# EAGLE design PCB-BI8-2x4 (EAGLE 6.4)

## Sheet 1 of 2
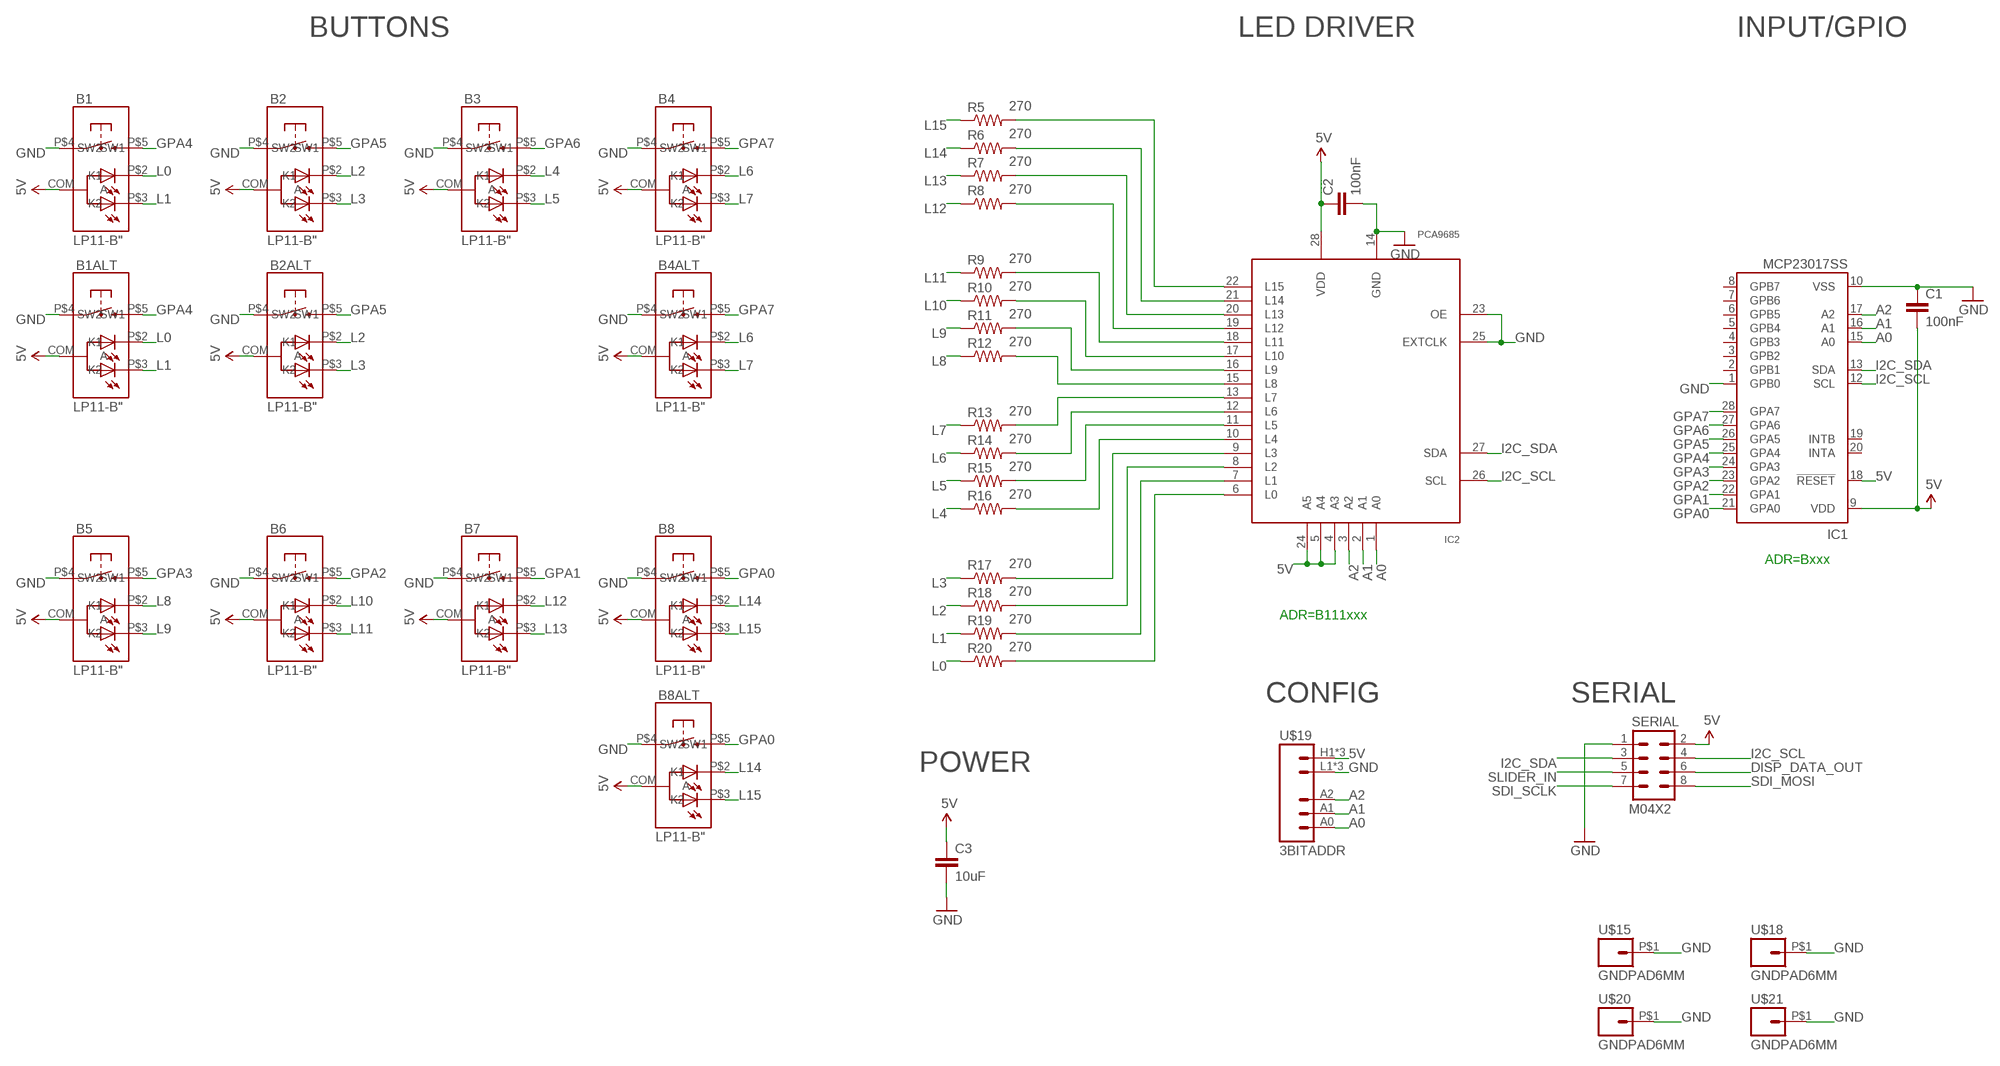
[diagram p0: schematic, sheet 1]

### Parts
B1  LP11-B"  [LP11]
B1ALT  LP11-B"  [LP11]
B2  LP11-B"  [LP11]
B2ALT  LP11-B"  [LP11]
B3  LP11-B"  [LP11]
B4  LP11-B"  [LP11]
B4ALT  LP11-B"  [LP11]
B5  LP11-B"  [LP11]
B6  LP11-B"  [LP11]
B7  LP11-B"  [LP11]
B8  LP11-B"  [LP11]
B8ALT  LP11-B"  [LP11]
C1  100nF  CAP0603-CAP  [0603-CAP]
C2  100nF  CAP0603-CAP  [0603-CAP]
C3  10uF  CAP0805  [0805]
IC1  MCP23017SS  [SSOP28]
IC2  PCA9685  [TSSOP28]
R5  270  RESISTOR0603-RES  [0603-RES]
R6  270  RESISTOR0603-RES  [0603-RES]
R7  270  RESISTOR0603-RES  [0603-RES]
R8  270  RESISTOR0603-RES  [0603-RES]
R9  270  RESISTOR0603-RES  [0603-RES]
R10  270  RESISTOR0603-RES  [0603-RES]
R11  270  RESISTOR0603-RES  [0603-RES]
R12  270  RESISTOR0603-RES  [0603-RES]
R13  270  RESISTOR0603-RES  [0603-RES]
R14  270  RESISTOR0603-RES  [0603-RES]
R15  270  RESISTOR0603-RES  [0603-RES]
R16  270  RESISTOR0603-RES  [0603-RES]
R17  270  RESISTOR0603-RES  [0603-RES]
R18  270  RESISTOR0603-RES  [0603-RES]
R19  270  RESISTOR0603-RES  [0603-RES]
R20  270  RESISTOR0603-RES  [0603-RES]
SERIAL  M04X2  [2X4]
U$15  GNDPAD6MM  [3.2MMPAD6MM]
U$18  GNDPAD6MM  [3.2MMPAD6MM]
U$19  3BITADDR  [3BITADDR]
U$20  GNDPAD6MM  [3.2MMPAD6MM]
U$21  GNDPAD6MM  [3.2MMPAD6MM]

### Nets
5V [Power]: B1.COM(A) B1ALT.COM(A) B2.COM(A) B2ALT.COM(A) B3.COM(A) B4.COM(A) B4ALT.COM(A) B5.COM(A) B6.COM(A) B7.COM(A) B8.COM(A) B8ALT.COM(A) C1.2 C2.1 C3.1 IC1.9(VDD) IC1.18(!RESET) IC2.4(A3) IC2.5(A4) IC2.24(A5) IC2.28(VDD) SERIAL.2 U$19.H1(VCC) U$19.H2(VCC) U$19.H3(VCC)
A0: IC1.15(A0) IC2.1(A0) U$19.A0
A1: IC1.16(A1) IC2.2(A1) U$19.A1
A2: IC1.17(A2) IC2.3(A2) U$19.A2
DISP_DATA_OUT: SERIAL.6
GND [Power]: B1.P$4(SW1) B1ALT.P$4(SW1) B2.P$4(SW1) B2ALT.P$4(SW1) B3.P$4(SW1) B4.P$4(SW1) B4ALT.P$4(SW1) B5.P$4(SW1) B6.P$4(SW1) B7.P$4(SW1) B8.P$4(SW1) B8ALT.P$4(SW1) C1.1 C2.2 C3.2 IC1.1(GPB0) IC1.10(VSS) IC2.14(GND) IC2.23(OE) IC2.25(EXTCLK) SERIAL.1 U$15.P$1 U$18.P$1 U$19.L1(GND) U$19.L2(GND) U$19.L3(GND) U$20.P$1 U$21.P$1
GPA0: B8.P$5(SW2) B8ALT.P$5(SW2) IC1.21(GPA0)
GPA1: B7.P$5(SW2) IC1.22(GPA1)
GPA2: B6.P$5(SW2) IC1.23(GPA2)
GPA3: B5.P$5(SW2) IC1.24(GPA3)
GPA4: B1.P$5(SW2) B1ALT.P$5(SW2) IC1.25(GPA4)
GPA5: B2.P$5(SW2) B2ALT.P$5(SW2) IC1.26(GPA5)
GPA6: B3.P$5(SW2) IC1.27(GPA6)
GPA7: B4.P$5(SW2) B4ALT.P$5(SW2) IC1.28(GPA7)
I2C_SCL: IC1.12(SCL) IC2.26(SCL) SERIAL.4
I2C_SDA: IC1.13(SDA) IC2.27(SDA) SERIAL.3
L0: B1.P$2(K1) B1ALT.P$2(K1) R20.1
L1: B1.P$3(K2) B1ALT.P$3(K2) R19.1
L2: B2.P$2(K1) B2ALT.P$2(K1) R18.1
L3: B2.P$3(K2) B2ALT.P$3(K2) R17.1
L4: B3.P$2(K1) R16.1
L5: B3.P$3(K2) R15.1
L6: B4.P$2(K1) B4ALT.P$2(K1) R14.1
L7: B4.P$3(K2) B4ALT.P$3(K2) R13.1
L8: B5.P$2(K1) R12.1
L9: B5.P$3(K2) R11.1
L10: B6.P$2(K1) R10.1
L11: B6.P$3(K2) R9.1
L12: B7.P$2(K1) R8.1
L13: B7.P$3(K2) R7.1
L14: B8.P$2(K1) B8ALT.P$2(K1) R6.1
L15: B8.P$3(K2) B8ALT.P$3(K2) R5.1
N$4: IC2.13(L7) R13.2
N$5: IC2.12(L6) R14.2
N$7: IC2.11(L5) R15.2
N$9: IC2.10(L4) R16.2
N$10: IC2.9(L3) R17.2
N$11: IC2.8(L2) R18.2
N$12: IC2.7(L1) R19.2
N$19: IC2.6(L0) R20.2
N$20: IC2.15(L8) R12.2
N$21: IC2.16(L9) R11.2
N$22: IC2.17(L10) R10.2
N$23: IC2.18(L11) R9.2
N$24: IC2.19(L12) R8.2
N$25: IC2.20(L13) R7.2
N$26: IC2.21(L14) R6.2
N$27: IC2.22(L15) R5.2
SDI_MOSI: SERIAL.8
SDI_SCLK: SERIAL.7
SLIDER_IN: SERIAL.5
Unconnected: IC1.2(GPB1) IC1.3(GPB2) IC1.4(GPB3) IC1.5(GPB4) IC1.6(GPB5) IC1.7(GPB6) IC1.8(GPB7) IC1.19(INTB) IC1.20(INTA)

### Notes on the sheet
- BUTTONS | LED DRIVER | INPUT/GPIO
- ADR=Bxxx
- ADR=B111xxx
- CONFIG | SERIAL
- POWER

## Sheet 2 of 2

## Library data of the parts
B1 B1ALT B2 B2ALT B3 B4 B4ALT B5-B8 B8ALT = SKAARHOJ:LP11-B
C1-C3 = SparkFun:CAP: Capacitor
IC1 = microchip:MCP23017: http://ww1.microchip.com/downloads/en/DeviceDoc/21952a.pdf Source: http://ww1.microchip.com/downloads/en/DeviceDoc/21952a.pdf; MF: MICROCHIP; MPN: MCP23017-E/SS; OC_FARNELL: 1467674; OC_NEWARK: 31K2960
IC2 = wsmith:PCA9685
R5-R20 = SparkFun:RESISTOR: Resistor
SERIAL = SparkFun:M04X2
U$15 U$18 U$20 U$21 = SKAARHOJ:GNDPAD
U$19 = SKAARHOJ:3BITADDR

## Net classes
0 default: width 0.203 mm, drill 0.406 mm, clearance 0.203 mm
1 Power: width 0.406 mm, drill 0.61 mm, clearance 0.203 mm

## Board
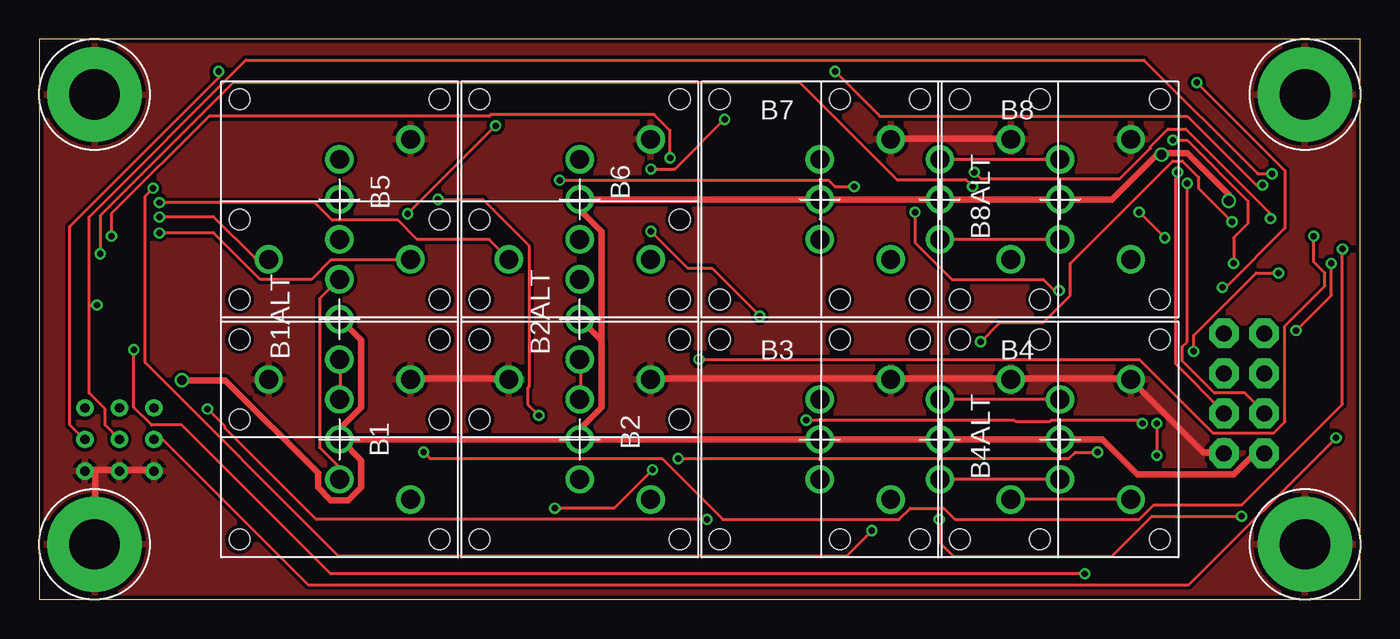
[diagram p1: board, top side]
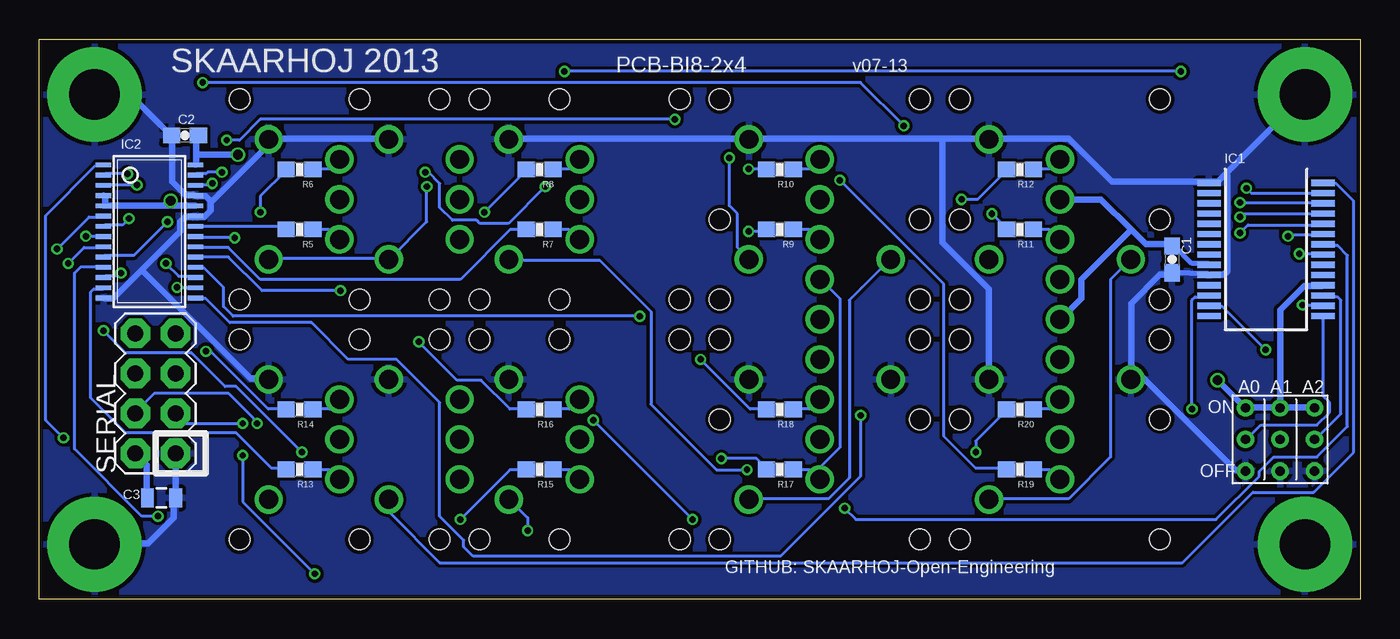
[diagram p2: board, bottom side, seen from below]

Size 83.82 x 35.56 mm. Coordinates in mm from the lower left corner, seen from the top.
Outline: 0,0 83.82,0 83.82,35.56 0,35.56 0,0
Copper layers (1*16): Top 0.035mm / dielectric 1.5mm / Bottom 0.035mm
Design rules "Fusion_eagle_rule_v1.1": minimum track width 6mil, minimum drill 12mil, track to track 6mil, track to pad 6mil, pad to pad 6mil, via to via 6mil, smd to smd 0mil, copper to edge 10mil, drill to drill 10mil, minimum pad ring 10mil, minimum via ring 6mil, stop-mask expansion 2mil, vias tented up to drill 100mil, thermal gap 10mil

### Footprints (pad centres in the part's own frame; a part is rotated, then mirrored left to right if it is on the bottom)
LP11 = drill 1.2: COM 0,0; P$2 0,2.54; P$3 0,-2.54; P$4 4.5,3.81; P$5 4.5,-3.81 | hole 1.3: -6.35,6.35; 6.35,6.35; 6.35,-6.35; -6.35,-6.35
0603-CAP = smd 1.1 x 1: 1 -0.85,0; 2 0.85,0
0805 = smd 0.8 x 1.2: 1 -0.9,0; 2 0.9,0
SSOP28 = smd 0.4 x 1.5: 1 -4.225,-3.625; 2 -3.575,-3.625; 3 -2.925,-3.625; 4 -2.275,-3.625; 5 -1.625,-3.625; 6 -0.975,-3.625; 7 -0.325,-3.625; 8 0.325,-3.625; 9 0.975,-3.625; 10 1.625,-3.625; 11 2.275,-3.625; 12 2.925,-3.625; 13 3.575,-3.625; 14 4.225,-3.625; 15 4.225,3.625; 16 3.575,3.625; 17 2.925,3.625; 18 2.275,3.625; 19 1.625,3.625; 20 0.975,3.625; 21 0.325,3.625; 22 -0.325,3.625; 23 -0.975,3.625; 24 -1.625,3.625; 25 -2.275,3.625; 26 -2.925,3.625; 27 -3.575,3.625; 28 -4.225,3.625
TSSOP28 = smd 0.305 x 0.991: 1 -4.225,-2.918; 2 -3.575,-2.918; 3 -2.925,-2.918; 4 -2.275,-2.918; 5 -1.625,-2.918; 6 -0.975,-2.918; 7 -0.325,-2.918; 8 0.325,-2.918; 9 0.975,-2.918; 10 1.625,-2.918; 11 2.275,-2.918; 12 2.925,-2.918; 13 3.575,-2.918; 14 4.225,-2.918; 15 4.225,2.918; 16 3.575,2.918; 17 2.925,2.918; 18 2.275,2.918; 19 1.625,2.918; 20 0.975,2.918; 21 0.325,2.918; 22 -0.325,2.918; 23 -0.975,2.918; 24 -1.625,2.918; 25 -2.275,2.918; 26 -2.925,2.918; 27 -3.575,2.918; 28 -4.225,2.918
0603-RES = smd 1.1 x 1: 1 -0.85,0; 2 0.85,0
2X4 = drill 1.016 pad 1.88 octagon: 1 -3.81,-1.27; 2 -3.81,1.27; 3 -1.27,-1.27; 4 -1.27,1.27; 5 1.27,-1.27; 6 1.27,1.27; 7 3.81,-1.27; 8 3.81,1.27
3.2MMPAD6MM = drill 3.2 pad 6: P$1 0,0
3BITADDR = drill 0.6: A0 -2.2,0; A1 0,0; A2 2.2,0; H1 -2.2,2; H2 0,2; H3 2.2,2; L1 -2.2,-2; L2 0,-2; L3 2.2,-2

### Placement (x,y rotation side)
B1  19.05,10.16 0 top
B1ALT  19.05,17.78 180 top
B2  34.29,10.16 0 top
B2ALT  34.29,17.78 180 top
B3  49.53,10.16 0 top
B4  64.77,10.16 0 top
B4ALT  57.15,10.16 0 top
B5  19.05,25.4 0 top
B6  34.29,25.4 0 top
B7  49.53,25.4 0 top
B8  64.77,25.4 0 top
B8ALT  57.15,25.4 0 top
C1  11.94,21.59 90 bottom
C2  74.57,29.46 180 bottom
C3  76.07,6.45 0 bottom
IC1  5.97,22.23 270 bottom
IC2  76.83,23.37 270 bottom
R5  67.31,23.5 180 bottom
R6  67.31,27.3 180 bottom
R7  52.07,23.5 180 bottom
R8  52.07,27.3 180 bottom
R9  36.83,23.5 180 bottom
R10  36.83,27.3 180 bottom
R11  21.59,23.5 180 bottom
R12  21.59,27.3 180 bottom
R13  67.31,8.26 180 bottom
R14  67.31,12.06 180 bottom
R15  52.07,8.26 180 bottom
R16  52.07,12.06 180 bottom
R17  36.83,8.26 180 bottom
R18  36.83,12.06 180 bottom
R19  21.59,8.26 180 bottom
R20  21.59,12.06 180 bottom
SERIAL  76.45,13.08 90 bottom
U$15  3.5,3.5 0 top
U$18  80.32,3.5 0 top
U$19  5.08,10.16 0 bottom
U$20  3.5,32.06 0 top
U$21  80.32,32.06 0 top

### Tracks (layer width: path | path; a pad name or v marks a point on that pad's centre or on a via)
5V  (via drill 0.61)
  Top 0.406: v75.49,25.3 75.49,25.7 72.85,28.35 71.32,28.35 v71.22,28.25 70.92,28.25 68.07,25.4 B8.COM B8ALT.COM B7.COM B6.COM 34.34,25.4 34.34,24.69 35.66,23.37 35.66,16.66 35.56,16.56 | SERIAL.2 77.72,9.25 77.11,9.25 75.79,7.92 69.7,7.92 67.46,10.16 B4.COM B4ALT.COM B3.COM B2.COM | 35.56,16.56 34.34,17.78 B2ALT.COM | 35.56,16.56 35.66,16.46 35.66,12.19 34.34,10.87 34.34,10.16 B2.COM | B1.COM 19.1,10.16 19.1,10.87 20.42,12.19 20.42,16.46 19.1,17.78 B1ALT.COM | v9.04,13.92 11.79,13.92 17.68,8.03 17.68,7.11 18.49,6.3 19.61,6.3 20.42,7.11 20.42,8.84 19.2,10.06 B1.COM | B1.COM B2.COM
  Bottom 0.305: IC1.9 9.68,21.34 10.67,21.34 11.77,22.44 C1.2
  Bottom 0.406: 79.65,24.99 75.49,24.99 | 75.49,24.99 73.97,24.99 IC2.24 | 79.65,24.99 IC2.5 | 79.65,24.99 79.65,25.6 IC2.4 | 73.86,28.25 73.86,29.36 73.76,29.46 C2.1 | 73.86,28.25 73.86,27.64 IC2.28 | v71.22,28.25 73.86,28.25 | v75.49,25.3 75.49,24.99 | C3.1 77.01,6.5 77.01,8.53 77.72,9.25 SERIAL.2 | U$19.H2 5.08,18.39 3.56,19.91 2.44,19.91 IC1.18 | U$19.H3 2.95,12.19 4.98,12.19 U$19.H2 | U$19.H2 5.28,12.19 7.21,12.19 U$19.H1 7.42,12.29 v9.04,13.92 | 14.53,23.47 16.46,25.4 B5.COM | 14.53,23.47 13.61,22.55 11.99,22.55 C1.2 | 14.53,23.47 17.68,20.32 17.68,19.1 19,17.78 B1ALT.COM
A0  (via drill 0.41)
  Top 0.203: v82.3,10.26 72.95,0.91 17.07,0.91 7.82,10.16 U$19.A0
  Bottom 0.203: v82.3,10.26 83.41,11.38 83.41,24.38 80.26,27.53 79.76,27.53 IC2.1 | IC1.15 2.34,17.98 2.34,12.9 1.93,12.5 1.93,11.89 2.74,11.07 6.3,11.07 7.21,10.16 U$19.A0
A1  (via drill 0.41)
  Top 0.203: v78.23,27.03 77.32,27.03 70.1,34.24 13.11,34.24 3.15,24.28 3.15,18.69 | 3.15,18.69 3.15,13.11 4.17,12.09 4.17,11.07 U$19.A1 | 3.15,18.69 v3.66,18.69
  Bottom 0.203: v78.23,27.03 79.65,27.03 IC2.2 | v3.66,18.69 2.44,18.69 IC1.16
A2  (via drill 0.41)
  Top 0.203: v77.62,26.31 77.22,26.31 72.85,30.68 53.34,30.68 v50.49,33.53 | v11.38,33.53 11.38,33.12 1.93,23.67 1.93,11.07 2.85,10.16 U$19.A2
  Bottom 0.203: v77.62,26.31 79.65,26.31 IC2.3 | v11.38,33.53 v50.49,33.53 | IC1.17 2.34,19.2 1.42,19.2 1.22,19 1.22,11.79 2.85,10.16 U$19.A2
GND
  Top 0.406: B2.P$4 38.81,14.02 53.95,14.02 B3.P$4 54.15,14.02 61.57,14.02 B4ALT.P$4 61.77,14.02 69.19,14.02 B4.P$4 69.39,13.82 73.86,9.35 75.18,9.35 SERIAL.1 | 3.56,8.23 5.08,8.23 U$19.L2 5.18,8.23 7.21,8.23 U$19.L1 | 3.56,8.23 2.95,8.23 U$19.L3 | 3.56,8.23 3.56,3.56 U$15.P$1 | B1.P$4 23.57,14.02 29.77,14.02 B2ALT.P$4 | B7.P$4 54.05,29.26 61.57,29.26 B8ALT.P$4
  Bottom 0.305: IC1.10 9.7,20.7 10.79,20.7 10.83,20.74 C1.1
  Bottom 0.406: SERIAL.1 75.18,6.5 C3.2 75.29,6.3 75.29,5.18 76.91,3.56 80.26,3.56 U$18.P$1 | U$20.P$1 8.53,27.03 | 8.53,27.03 9.04,26.52 9.55,26.52 IC1.1 9.75,26.52 15.75,26.52 18.49,29.26 23.37,29.26 B5.P$4 23.57,29.26 26.52,29.26 | IC1.10 9.45,20.62 8.64,20.62 8.43,20.83 8.43,26.92 8.53,27.03 | C1.1 11.99,20.62 12.7,20.62 14.53,18.8 14.53,14.02 B1ALT.P$4 14.43,14.73 7.92,8.23 7.32,8.23 U$19.L1 | 26.52,29.26 38.71,29.26 B6.P$4 38.91,29.26 53.95,29.26 B7.P$4 | 26.52,29.26 26.52,22.66 23.57,19.71 23.57,14.02 B1.P$4 | 72.95,25.3 72.95,24.69 73.36,24.28 73.86,24.28 IC2.23 74.07,24.28 74.57,24.28 74.88,23.98 74.88,23.37 77.32,20.93 | 72.95,25.3 73.25,25.6 73.86,25.6 IC2.25 74.07,25.7 74.57,25.7 75.39,26.52 75.39,29.46 C2.2 75.59,29.57 78.03,32 80.26,32 U$21.P$1 | 77.32,20.93 79.15,19.1 79.65,19.1 IC2.14 | 72.95,25.3 72.85,25.3 69.29,28.85 69.29,29.16 B8.P$4 69.09,29.26 61.67,29.26 B8ALT.P$4 | 77.32,20.93 70.41,14.02 69.29,14.02 B4.P$4
  pour Top: 0,0 83.82,0 83.82,35.56 0,35.56
  pour Bottom: 0,0 83.82,0 83.82,35.56 0,35.56
GPA0  (via drill 0.41)
  Top 0.203: v3.86,21.95 3.86,24.38 12.29,32.82 48.26,32.82 54.46,26.62 58.83,26.62 v59.23,26.21
  Bottom 0.203: v3.86,21.95 2.44,21.95 IC1.21 | v59.23,26.21 59.23,23.98 61.57,21.64 B8ALT.P$5 61.67,21.64 69.19,21.64 B8.P$5
GPA1  (via drill 0.41)
  Top 0.203: v32.72,5.79 36.47,5.79 v38.91,8.23
  Bottom 0.203: v32.72,5.79 32,5.08 9.14,5.08 6.4,7.82 6.4,8.13 5.49,9.04 2.74,9.04 0.81,10.97 0.81,21.84 1.42,22.45 2.34,22.45 IC1.22 | v38.91,8.23 40.84,8.23 45.01,12.39 45.01,18.29 48.26,21.54 53.95,21.54 B7.P$5
GPA2  (via drill 0.41)
  Top 0.203: v4.57,23.06 4.57,24.49 10.77,30.68 28.55,30.68 28.65,30.79 39.01,30.79 40.03,29.77 v40.03,28.04
  Bottom 0.203: v4.57,23.06 4.47,23.16 2.44,23.16 IC1.23 | v40.03,28.04 40.03,24.99 39.52,24.49 39.52,22.35 38.81,21.64 B6.P$5
GPA3  (via drill 0.41)
  Top 0.203: v7.62,23.27 11.07,23.27 14.02,20.32 17.27,20.32 18.49,21.54 23.47,21.54 B5.P$5
  Bottom 0.203: v7.62,23.27 7.11,23.77 2.44,23.77 IC1.24
GPA4  (via drill 0.41)
  Top 0.203: v7.62,24.28 11.07,24.28 13.72,21.64 14.53,21.64 B1ALT.P$5
  Bottom 0.203: v7.62,24.28 7.42,24.49 2.44,24.49 IC1.25 | B1.P$5 23.47,6.4 18.49,6.4 15.85,9.04 15.85,20.32 14.63,21.54 B1ALT.P$5
GPA5  (via drill 0.41)
  Top 0.203: v7.62,25.2 17.48,25.2 18.59,24.08 22.76,24.08 23.98,22.86 28.55,22.86 29.77,21.64 B2ALT.P$5
  Bottom 0.203: v7.62,25.2 2.44,25.2 IC1.26 | B2.P$5 38.71,6.4 33.73,6.4 32.41,7.72 32.41,19 29.87,21.54 B2ALT.P$5
GPA6  (via drill 0.41)
  Top 0.203: v7.21,26.11 6.71,25.6 6.71,15.04 19,2.74 51.21,2.74 v52.83,4.37
  Bottom 0.203: v7.21,26.11 6.91,25.81 2.44,25.81 IC1.27 | v52.83,4.37 52.83,5.18 53.95,6.3 B3.P$5
GPA7
  Top 0.203: B4.P$5 69.19,6.4 61.67,6.4 B4ALT.P$5
  Bottom 0.203: IC1.28 2.34,26.42 1.52,26.42 0.41,25.3 0.41,9.35 2.95,6.81 6.81,6.81 11.28,2.34 58.42,2.34 61.57,5.49 61.57,6.3 B4ALT.P$5
I2C_SCL  (via drill 0.41)
  Top 0.203: v72.85,26.42 72.85,16.36 72.54,16.05 72.54,15.14 74.57,13.11 76.5,13.11 77.72,11.89 SERIAL.4 | v10.67,12.09 11.79,10.97 11.79,10.87 17.58,5.08 v42.37,5.08 | v48.67,11.38 61.87,11.38 61.98,11.28 64.11,11.28 64.21,11.38 69.8,11.38 v70,11.18
  Bottom 0.203: v72.85,26.42 72.95,26.31 73.86,26.31 IC2.26 | v10.67,12.09 10.67,19 10.46,19.2 9.65,19.2 IC1.12 | v48.67,11.38 v42.37,5.08 | v70,11.18 70.21,11.38 70.21,11.48 71.83,13.11 76.5,13.11 77.72,11.89 SERIAL.4
I2C_SDA  (via drill 0.41)
  Top 0.203: v72.24,27.13 72.24,26.82 72.14,26.72 72.14,14.94 75.18,11.89 SERIAL.3 | v5.99,15.85 5.99,12.19 7.11,11.07 9.04,11.07 18.49,1.63 v66.34,1.63 | v70.92,11.18 v70.92,9.14
  Bottom 0.203: v72.24,27.13 73.15,27.13 73.25,27.03 73.86,27.03 IC2.27 | v5.99,15.85 8.74,18.59 9.55,18.59 IC1.13 | v66.34,1.63 70.92,6.2 v70.92,9.14 | v70.92,11.18 74.57,11.18 75.18,11.79 SERIAL.3
L0
  Top 0.203: B1.P$2 19.1,12.7 19.1,15.24 B1ALT.P$2
  Bottom 0.203: R20.1 20.73,12.09 19.71,12.09 19.1,12.7 B1.P$2
L1
  Top 0.203: B1.P$3 19,7.62 19,8.43 17.78,9.65 17.78,19.1 19,20.32 B1ALT.P$3
  Bottom 0.203: R19.1 20.73,8.23 19.71,8.23 19.1,7.62 B1.P$3
L2
  Top 0.203: B2.P$2 34.34,12.7 34.34,15.24 B2ALT.P$2
  Bottom 0.203: R18.1 35.97,12.09 34.95,12.09 34.34,12.7 B2.P$2
L3
  Bottom 0.203: R17.1 35.97,8.23 34.95,8.23 34.34,7.62 B2.P$3 34.65,8.03 33.02,9.65 33.02,19.1 34.24,20.32 B2ALT.P$3
L4
  Bottom 0.203: R16.1 51.21,12.09 50.19,12.09 49.58,12.7 B3.P$2
L5
  Bottom 0.203: R15.1 51.21,8.23 50.19,8.23 49.58,7.62 B3.P$3
L6
  Top 0.203: B4.P$2 B4ALT.P$2
  Bottom 0.203: R14.1 66.45,12.09 65.43,12.09 64.82,12.7 B4.P$2
L7
  Top 0.203: B4.P$3 B4ALT.P$3
  Bottom 0.203: R13.1 66.45,8.23 65.43,8.23 64.82,7.62 B4.P$3
L8
  Bottom 0.203: R12.1 20.73,27.33 19.71,27.33 19.1,27.94 B5.P$2
L9
  Bottom 0.203: R11.1 20.73,23.47 19.71,23.47 19.1,22.86 B5.P$3
L10
  Bottom 0.203: R10.1 35.97,27.33 34.95,27.33 34.34,27.94 B6.P$2
L11
  Bottom 0.203: R9.1 35.97,23.47 34.95,23.47 34.34,22.86 B6.P$3
L12
  Bottom 0.203: R8.1 51.21,27.33 50.19,27.33 49.58,27.94 B7.P$2
L13
  Bottom 0.203: R7.1 51.21,23.47 50.19,23.47 49.58,22.86 B7.P$3
L14
  Top 0.203: B8.P$2 B8ALT.P$2
  Bottom 0.203: R6.1 66.45,27.33 65.43,27.33 64.82,27.94 B8.P$2
L15
  Top 0.203: B8.P$3 B8ALT.P$3
  Bottom 0.203: R5.1 66.45,23.47 65.43,23.47 64.82,22.86 B8.P$3
N$4
  Bottom 0.203: IC2.13 79.76,19.71 80.37,19.71 80.57,19.51 80.57,12.8 78.33,10.57 71.32,10.57 69.09,8.33 68.17,8.33 R13.2
N$5  (via drill 0.41)
  Top 0.203: v78.64,20.73 77.22,20.73 73.25,16.76 v73.25,15.75
  Bottom 0.203: v78.64,20.73 78.84,20.52 79.65,20.52 IC2.12 | v73.25,15.75 72.95,15.75 69.29,12.09 68.17,12.09 R14.2
N$7  (via drill 0.41)
  Top 0.203: v76.3,5.28 70.61,5.28 68.07,2.74 58.01,2.74 57.1,3.66 v57.1,5.08
  Bottom 0.203: v76.3,5.28 77.32,5.28 81.58,9.55 81.58,20.73 81.18,21.13 79.76,21.13 IC2.11 | v57.1,5.08 53.95,8.23 52.93,8.23 R15.2
N$9  (via drill 0.41)
  Top 0.203: v75.69,23.98 73.56,26.11 73.56,26.82 72.54,27.84 71.93,27.84 65.43,21.34 65.43,19.3 63.7,17.58 60.96,17.58 v59.74,16.36
  Bottom 0.203: v75.69,23.98 77.83,21.84 79.65,21.84 IC2.10 | v59.74,16.36 57.3,13.92 55.78,13.92 53.95,12.09 52.93,12.09 R16.2
N$10  (via drill 0.41)
  Top 0.203: v81.99,21.34 81.99,19.3 v79.76,17.07 | v67.16,9.35 65.73,9.35 65.33,8.94 v40.54,8.94
  Bottom 0.203: v81.99,21.34 80.97,22.35 79.76,22.35 IC2.9 | v79.76,17.07 78.33,15.65 74.17,15.65 72.03,13.51 71.32,13.51 v67.16,9.35 | v40.54,8.94 38.3,8.94 37.69,8.33 R17.2
N$11  (via drill 0.41)
  Top 0.203: v80.87,23.06 80.87,21.44 81.58,20.73 81.58,19.91 79.05,17.37 79.05,11.28 78.33,10.57 74.47,10.57 69.8,15.24 v41.86,15.24
  Bottom 0.203: v80.87,23.06 79.76,23.06 IC2.8 | v41.86,15.24 38.71,12.09 37.69,12.09 R18.2
N$12  (via drill 0.41)
  Top 0.203: v78.13,24.18 78.13,24.49 72.75,29.87 71.63,29.87 70.51,28.75 70.51,28.65 68.58,26.72 59.74,26.72 v59.33,27.13 | v51.71,26.21 50.49,26.21 50.09,26.62 v33.02,26.62
  Bottom 0.203: v78.13,24.18 78.54,23.77 79.65,23.77 IC2.7 | v59.33,27.13 59.13,27.13 58.42,26.42 58.42,24.89 57.61,24.08 56.08,24.08 55.88,23.88 54.05,23.88 v51.71,26.21 | v33.02,26.62 26.42,20.02 26.42,10.36 24.38,8.33 22.45,8.33 R19.2
N$19  (via drill 0.41)
  Top 0.203: v82.7,22.25 82.7,12.39 76.3,5.99 70.71,5.99 69.8,5.08 58.12,5.08 57.4,5.79 55.27,5.79 54.56,5.08 43.38,5.08 39.52,8.94 24.79,8.94 v24.38,9.35
  Bottom 0.203: v82.7,22.25 80.67,24.28 79.76,24.28 IC2.6 | v24.38,9.35 24.38,10.06 22.45,11.99 R20.2
N$20  (via drill 0.41)
  Top 0.203: v31.7,11.68 30.99,12.39 30.99,13.41 31.09,13.51 31.09,22.45 28.14,25.4 v25.3,25.4
  Bottom 0.203: v31.7,11.68 31.7,7.82 36.78,2.74 56.29,2.74 56.9,3.35 56.9,3.76 58.42,5.28 58.42,12.5 61.16,15.24 64.21,15.24 66.55,17.58 71.73,17.58 73.25,19.1 73.86,19.1 IC2.15 | v25.3,25.4 24.28,25.4 22.45,27.23 R12.2
N$21  (via drill 0.41)
  Top 0.203: v75.08,19.81 75.29,19.81 79.05,23.57 79.05,27.23 v73.46,32.82 | v23.37,24.49 v28.96,30.07
  Bottom 0.203: v75.08,19.81 73.97,19.81 IC2.16 | v73.46,32.82 31.7,32.82 v28.96,30.07 | v23.37,24.49 22.45,23.57 R11.2
N$22  (via drill 0.41)
  Top 0.203: v75.79,21.34 75.79,22.96 76.71,23.88 76.71,25.3 72.85,29.16 v71.93,29.16 | v43.48,30.48 40.34,27.33 v38.81,27.33
  Bottom 0.203: v75.79,21.34 74.98,20.52 73.97,20.52 IC2.17 | v71.93,29.16 71.12,29.16 69.8,30.48 v43.48,30.48 | v38.81,27.33 37.69,27.33 R10.2
N$23  (via drill 0.41)
  Top 0.203: v45.72,17.98 42.67,21.03 41.15,21.03 v38.81,23.37
  Bottom 0.203: v45.72,17.98 71.53,17.98 72.14,18.59 72.14,19.81 73.36,21.03 73.86,21.03 IC2.18 | v38.81,23.37 37.8,23.37 37.69,23.47 R9.2
N$24  (via drill 0.41)
  Top 0.203: v64.72,19.61 64.41,19.61 63.7,20.32 57.91,20.32 55.58,22.66 v55.58,24.59
  Bottom 0.203: v64.72,19.61 69.7,19.61 71.83,21.74 73.86,21.74 IC2.19 | v55.58,24.59 52.93,27.23 R8.2
N$25
  Bottom 0.203: IC2.20 73.86,22.35 71.83,22.35 69.8,20.32 57.1,20.32 53.95,23.47 52.93,23.47 R7.2
N$26  (via drill 0.41)
  Top 0.203: v69.8,24.59 v71.42,22.96
  Bottom 0.203: v71.42,22.96 73.86,22.96 IC2.21 | v69.8,24.59 69.8,25.6 68.17,27.23 R6.2
N$27
  Bottom 0.203: IC2.22 73.86,23.67 68.28,23.67 68.17,23.57 R5.2

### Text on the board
_bsilk: v07-13 | PCB-BI8-2x4 | SKAARHOJ 2013 | GITHUB: SKAARHOJ-Open-Engineering

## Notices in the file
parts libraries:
SparkFun: Licensing: CC v3.0 Share-Alike You are welcome to use this library for commercial purposes.
